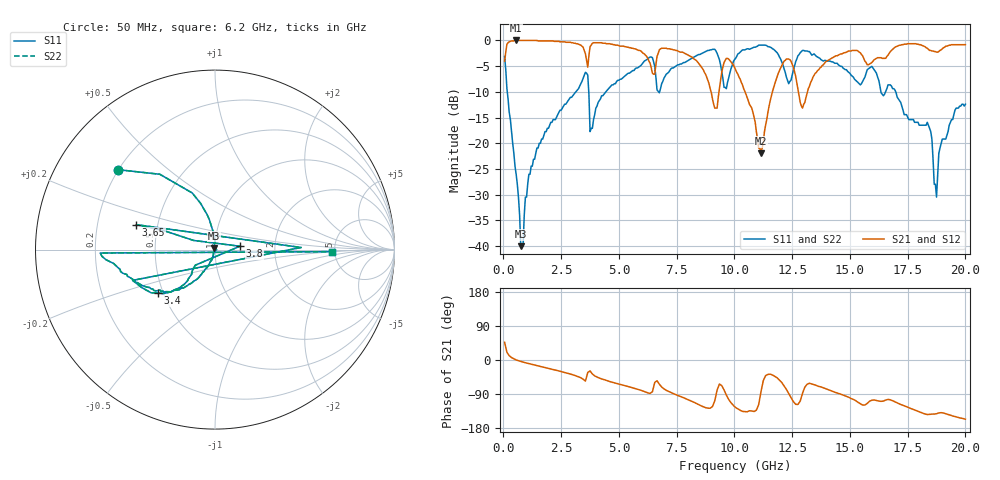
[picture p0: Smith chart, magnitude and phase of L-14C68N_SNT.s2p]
#	mhz	s	ma	r	50
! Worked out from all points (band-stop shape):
!   400 points, 50 MHz to 20 GHz, reference 50 ohm
!   highest |S21| = 0.00 dB at 550 MHz (marker M1); lowest = -21.9 dB at 11.15 GHz (marker M2)
!   |S21| within 3 dB of the highest: 79.06 MHz to 3.565 GHz (3.486 GHz wide, 191 % of centre); 16.62 GHz to end of sweep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
!   lowest |S11| = -40.0 dB at 750 MHz (marker M3), VSWR 1.02, Z = 49.6 + j0.912 ohm
!   |S11| at or under -10 dB: 165.7 MHz to 3.131 GHz (2.966 GHz wide, 180 % of centre); 3.694 GHz to 4.431 GHz (737.5 MHz wide, 18.2 % of centre); 16.98 GHz to end of sweep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
!   |S22| runs from -40.0 to -0.9 dB; largest |S21 - S12| = 0
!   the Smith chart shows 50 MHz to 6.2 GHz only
!   S11 on the Smith chart (normalised r, x): 50 MHz: 0.20, +0.35; 3.4 GHz: 0.47, -0.27; 3.65 GHz: 0.38, +0.13; 3.8 GHz: 1.32, +0.05; 6.2 GHz: 4.71, -0.18
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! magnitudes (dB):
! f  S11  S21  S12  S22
! 50 MHz  -3.1  -4.0  -4.0  -3.1
! 550 MHz  -26.0  0.0  0.0  -26.0
! 750 MHz  -40.0  0.0  0.0  -40.0
! 1.45 GHz  -20.9  0.0  0.0  -20.9
! 3.4 GHz  -8.0  -1.1  -1.1  -8.0
! 3.65 GHz  -6.7  -5.2  -5.2  -6.7
! 3.8 GHz  -17.1  -0.9  -0.9  -17.1
! 6.2 GHz  -3.7  -3.1  -3.1  -3.7
! 6.7 GHz  -9.9  -2.5  -2.5  -9.9
! 8.35 GHz  -3.0  -3.9  -3.9  -3.0
! 9.15 GHz  -1.7  -13.2  -13.2  -1.7
! 9.65 GHz  -9.4  -3.5  -3.5  -9.4
! 10.05 GHz  -3.5  -5.7  -5.7  -3.5
! 11.15 GHz  -0.9  -21.9  -21.9  -0.9
! 12.15 GHz  -5.5  -4.0  -4.0  -5.5
! 12.95 GHz  -1.9  -13.2  -13.2  -1.9
! 13.35 GHz  -2.9  -7.7  -7.7  -2.9
! 16.7 GHz  -8.6  -2.5  -2.5  -8.6
! 18.35 GHz  -15.9  -1.5  -1.5  -15.9
! 18.75 GHz  -30.5  -2.3  -2.3  -30.5
! 19 GHz  -19.2  -1.6  -1.6  -19.2
! 20 GHz  -12.4  -0.8  -0.8  -12.4
